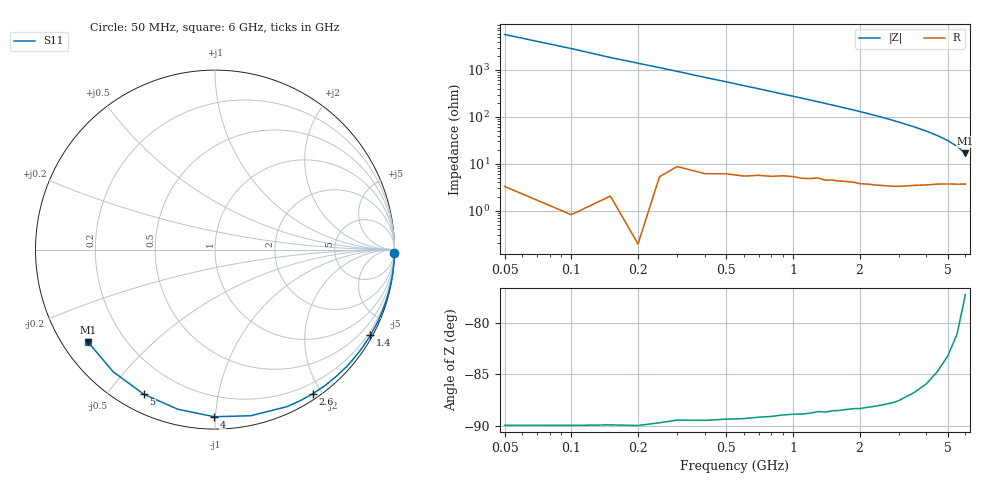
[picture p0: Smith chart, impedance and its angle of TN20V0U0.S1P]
! SIEMENS Discrete & RF Semiconductors
! BAS70-07W
! Si Schottky Diode in SOT343
! VR = 20 V
! S-Parameters:  February  1997
# GHz  S  MA  R  50
!  f  S11
! GHz  MAG  ANG
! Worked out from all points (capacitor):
!   34 points, 50 MHz to 6 GHz, reference 50 ohm
!   read as one part to ground: C = 556 fF near 50 MHz
!   lowest |Z| = 16.6 ohm at 6 GHz (marker M1)
!   S11 on the Smith chart (normalised r, x): 50 MHz: open; 1.4 GHz: 0.09, -3.88; 2.6 GHz: 0.07, -1.89; 4 GHz: 0.07, -0.99; 5 GHz: 0.07, -0.62; 6 GHz: 0.07, -0.32
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0.05  1 -1.0
0.2  1 -4.1
0.3  0.999 -6.1
0.4  0.9987 -8.2
0.6  0.9975 -12.3
0.7  0.9965 -14.3
0.8  0.9956 -16.4
0.9  0.9943 -18.5
1  0.9932 -20.5
1.1  0.9925 -22.6
1.2  0.9912 -24.7
1.4  0.9889 -28.9
1.5  0.9871 -31.1
1.6  0.986 -33.2
1.8  0.9831 -37.6
1.9  0.9816 -39.7
2  0.9808 -42.0
2.2  0.9774 -46.5
2.4  0.9742 -51.1
2.6  0.9705 -55.8
2.8  0.9667 -60.6
3  0.962 -65.5
3.5  0.9469 -77.8
4  0.9312 -90.3
4.5  0.9133 -103.1
5  0.8983 -116.2
5.5  0.8863 -129.8
6  0.8751 -144.0
